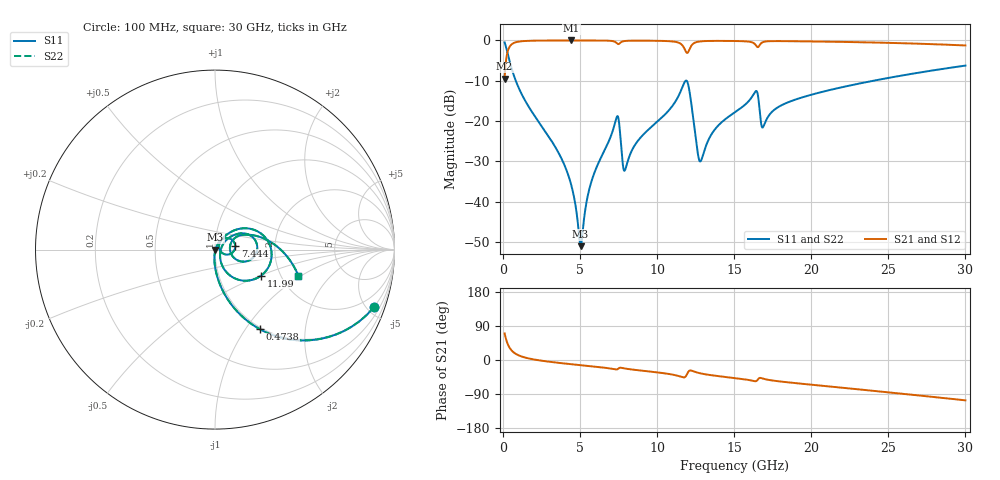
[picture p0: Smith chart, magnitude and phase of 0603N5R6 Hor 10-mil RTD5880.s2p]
# GHz S MA R 50
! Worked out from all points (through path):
!   3201 points, 100 MHz to 30 GHz, reference 50 ohm
!   highest |S21| = -0.02 dB at 4.436 GHz (marker M1); lowest = -9.5 dB at 100 MHz (marker M2)
!   group delay of S21, straight-line fit = 10.6 ps
!   lowest |S11| = -51.0 dB at 5.034 GHz (marker M3), VSWR 1.01, Z = 50.3 - j0.0798 ohm
!   |S11| at or under -10 dB: 823.9 MHz to 11.85 GHz (11.02 GHz wide, 174 % of centre); 11.91 GHz to 24.04 GHz (12.13 GHz wide, 67.5 % of centre)
!   |S22| runs from -51.0 to -0.5 dB; largest |S21 - S12| = 0
!   S11 on the Smith chart (normalised r, x): 100 MHz: 0.98, -5.56; 473.8 MHz: 0.98, -1.16; 7.444 GHz: 1.25, +0.05; 11.99 GHz: 1.60, -0.50; 30 GHz: 2.48, -0.95
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0.1  0.9423 -19.8  0.3346 70.2  0.3346 70.2  0.9423 -19.8
0.47375  0.5078 -60.7  0.8608 29.2  0.8608 29.2  0.5078 -60.7
1.324031  0.1954 -82.0  0.9794 7.7  0.9794 7.7  0.1954 -82.0
3.575875  0.04126 -94.3  0.9969 -7.4  0.9969 -7.4  0.04126 -94.3
4.4355  0.01585 -91.9  0.9973 -11.2  0.9973 -11.2  0.01585 -91.9
5.0335  0.00282 -16.3  0.9971 -13.7  0.9971 -13.7  0.00282 -16.3
5.089563  0.003122 10.3  0.9971 -13.9  0.9971 -13.9  0.003122 10.3
5.752969  0.01836 62.9  0.9964 -16.7  0.9964 -16.7  0.01836 62.9
7.444187  0.1147 10.2  0.9028 -23.9  0.9028 -23.9  0.1147 10.2
7.911375  0.02467 23.2  0.9825 -22.5  0.9825 -22.5  0.02467 23.2
10.06978  0.1008 52.6  0.987 -33.0  0.987 -33.0  0.1008 52.6
11.51806  0.2323 29.6  0.909 -43.9  0.909 -43.9  0.2323 29.6
11.98525  0.2955 -29.2  0.7049 -33.6  0.7049 -33.6  0.2955 -29.2
12.79816  0.0316 -10.4  0.971 -35.2  0.971 -35.2  0.0316 -10.4
13.68581  0.07628 39.8  0.9849 -41.1  0.9849 -41.1  0.07628 39.8
15.05  0.1289 38.0  0.9818 -47.7  0.9818 -47.7  0.1289 38.0
16.3955  0.2347 8.1  0.8745 -56.0  0.8745 -56.0  0.2347 8.1
16.89072  0.08546 12.0  0.956 -49.3  0.956 -49.3  0.08546 12.0
17.81575  0.1475 30.3  0.979 -55.9  0.979 -55.9  0.1475 30.3
20.03956  0.213 22.8  0.9697 -65.3  0.9697 -65.3  0.213 22.8
25.01978  0.343 3.3  0.9315 -85.4  0.9315 -85.4  0.343 3.3
30  0.4868 -17.4  0.8647 -106.4  0.8647 -106.4  0.4868 -17.4
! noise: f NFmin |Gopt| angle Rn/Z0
0.1  0.0003767  0.9367  0.6211  0.001326
3.417  0.004021  0.8093  9.368  0.004363
6.743  0.00994  0.8453  18.27  0.01331
10.06  0.01301  0.8266  27.08  0.01492
13.39  0.02055  0.853  35.92  0.02701
16.7  0.06102  0.9361  44.55  0.1823
20.03  0.01763  0.7615  52.54  0.01211
23.35  0.01938  0.7516  60.52  0.01182
26.67  0.02179  0.7508  68.35  0.01218
30  0.02454  0.754  75.98  0.01266
